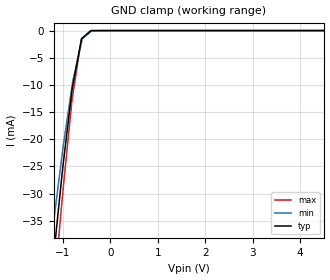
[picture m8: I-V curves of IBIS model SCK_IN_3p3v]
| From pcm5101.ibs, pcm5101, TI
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|   SCK_IN_3p3v
[Model]   SCK_IN_3p3v
Model_type   Input
Vinl = 0.99
Vinh = 2.31
|   typ   min   max
C_comp   1.009791957pF   0.990329415pF   1.034833107pF
[Voltage Range]   3.3   3   3.6
[Temperature Range]   27   105   -25
[Power Clamp Reference]   3.3   3   3.6
[GND Clamp Reference]   -0   -0   -0
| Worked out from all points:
|   GND clamp passes 1 mA (typ) near -0.54 V on its own axis
[GND Clamp]
|   Voltage   I(typ)   I(min)   I(max)
-3.3V     -526.2mA   -489.4mA   -552.7mA
-1.384V   -58.51mA   -49.12mA   -68.56mA
-1.208V   -42.45mA   -36.01mA   -49.95mA
-1.186V   -40.51mA   -34.34mA   -47.72mA
-1.01V    -25.63mA   -22.28mA   -30.25mA
-806.5mV  -10.7mA    -10.07mA   -12.62mA
-789.9mV  -9.929mA   -9.096mA   -11.67mA
-614.3mV  -1.741mA   -2.396mA   -1.618mA
-591.9mV  -1.349mA   -1.541mA   -1.436mA
-416.3mV  -55.3uA    -203.5uA   -6.682uA
-195.9mV  -8.324uA   -155.8nA   -2.963uA
6.6V      0A         0A         0A
[POWER Clamp]
|   Voltage   I(typ)   I(min)   I(max)
-3.3V     0A         0A         0A
0V        0A         0A         0A
6.6V      0A         0A         0A
